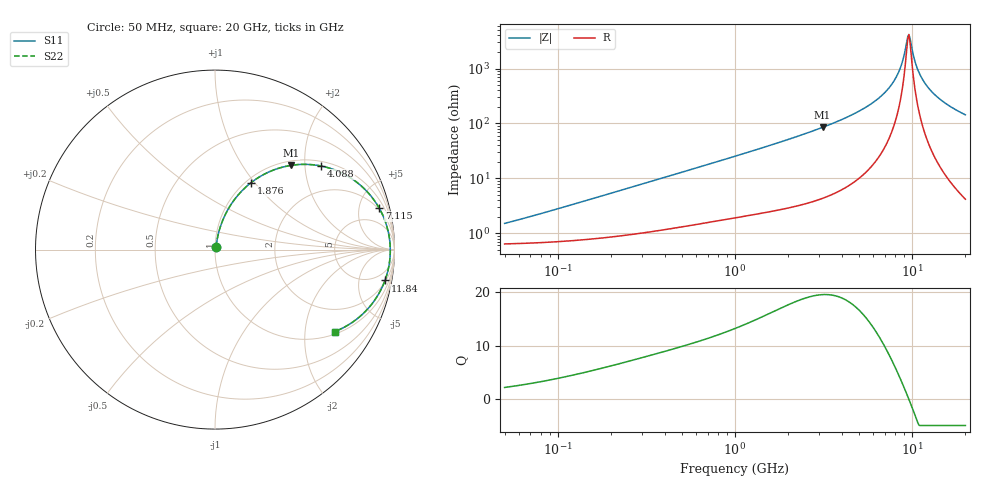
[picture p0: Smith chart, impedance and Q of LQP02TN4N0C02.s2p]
!Murata Part Number: LQP02TN4N0C02
!These Parameters are Measured in Series Mode Connection
!  o--[Z]--o
!Port1  Port2
!  o-------o
!Freq. Start=50[MHz] Stop=20[GHz], 401[Steps]
# Hz S RI R 50
!Freq.(Hz) S11(Real) S11(Imag) S21(Real) S21(Imag) S12(Real) S12(Imag) S22(Real) S22(Imag)
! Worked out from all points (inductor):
!   401 points, 50 MHz to 20 GHz, reference 50 ohm
!   read as one part in series: L = 4.32 nH near 73.81 MHz
!   highest Q = 19.6 at 3.122 GHz (marker M1), where L = 4.32 nH
!   self-resonance near 9.457 GHz
!   S11 on the Smith chart (normalised r, x): 50 MHz: 1.01, +0.03; 1.876 GHz: 1.06, +0.95; 4.088 GHz: 1.13, +2.42; 7.115 GHz: 1.81, +7.60; 11.84 GHz: 2, -11; 20 GHz: 1.08, -2.87
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5e7  0.00654 0.0135  0.9935 -0.0135  0.9935 -0.0135  0.00654 0.0135
1.364002e8  0.00883 0.0361  0.9912 -0.0361  0.9912 -0.0361  0.00883 0.0361
3.721004e8  0.02 0.0936  0.98 -0.0936  0.98 -0.0936  0.02 0.0936
1e9  0.0752 0.2285  0.9248 -0.2285  0.9248 -0.2285  0.0752 0.2285
1.875929e9  0.1994 0.3716  0.8006 -0.3716  0.8006 -0.3716  0.1994 0.3716
2.728004e9  0.3501 0.4518  0.6499 -0.4518  0.6499 -0.4518  0.3501 0.4518
3.121702e9  0.4222 0.469  0.5778 -0.469  0.5778 -0.469  0.4222 0.469
4.087748e9  0.5896 0.4661  0.4104 -0.4661  0.4104 -0.4661  0.5896 0.4661
5.598765e9  0.793 0.3729  0.207 -0.3729  0.207 -0.3729  0.793 0.3729
7.114996e9  0.9146 0.2315  0.0854 -0.2315  0.0854 -0.2315  0.9146 0.2315
7.442007e9  0.9312 0.1993  0.0688 -0.1993  0.0688 -0.1993  0.9312 0.1993
8.020766e9  0.9534 0.1427  0.0466 -0.1427  0.0466 -0.1427  0.9534 0.1427
8.516016e9  0.9661 0.0954  0.0339 -0.0954  0.0339 -0.0954  0.9661 0.0954
8.907419e9  0.9724 0.059  0.0276 -0.059  0.0276 -0.059  0.9724 0.059
9.316812e9  0.9759 0.0221  0.0241 -0.0221  0.0241 -0.0221  0.9759 0.0221
9.600142e9  0.9767 -0.00258  0.0233 0.00258  0.0233 0.00258  0.9767 -0.00258
9.892087e9  0.9762 -0.0273  0.0238 0.0273  0.0238 0.0273  0.9762 -0.0273
1.034674e10  0.9731 -0.0643  0.0269 0.0643  0.0269 0.0643  0.9731 -0.0643
1.066139e10  0.9694 -0.0887  0.0306 0.0887  0.0306 0.0887  0.9694 -0.0887
1.183995e10  0.947 -0.1719  0.053 0.1719  0.053 0.1719  0.947 -0.1719
1.460232e10  0.8619 -0.3179  0.1381 0.3179  0.1381 0.3179  0.8619 -0.3179
2e10  0.668 -0.4566  0.332 0.4566  0.332 0.4566  0.668 -0.4566
